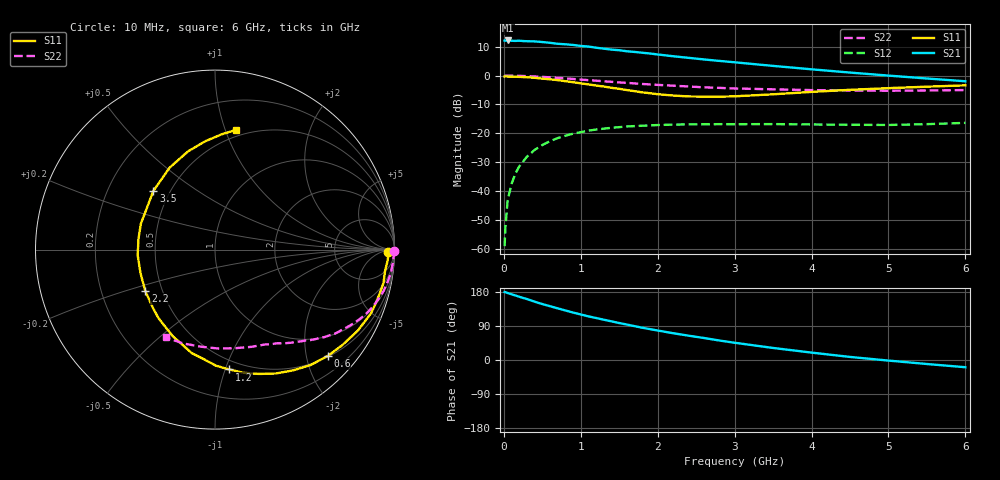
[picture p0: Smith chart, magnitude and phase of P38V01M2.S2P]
! SIEMENS Small Signal Semiconductors
! BFP181
! Si NPN RF Bipolar Junction Transistor in SOT143
! VCE = 8 V  IC = 1.2 mA
! Common Emitter S-Parameters:  March  1996
# GHz  S  MA  R  50
!  f  S11  S21  S12  S22
! GHz  MAG  ANG  MAG  ANG  MAG  ANG  MAG  ANG
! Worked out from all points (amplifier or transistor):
!   36 points, 10 MHz to 6 GHz, reference 50 ohm
!   highest |S21| = 12.2 dB at 50 MHz (marker M1)
!   |S21| within 3 dB of that: start of sweep to 1.347 GHz
!   unconditionally stable (mu >= 1): 3.037 GHz to end of sweep
!   at 250 MHz: K = 0.08, MSG = 20.9 dB, |S12| = -29.8 dB
!   at 1.4 GHz: K = 0.51, MSG = 13.6 dB, |S12| = -18.1 dB
!   at 6 GHz: K = 1.24, MAG = 4.3 dB, |S12| = -16.4 dB
!   S11 on the Smith chart (normalised r, x): 10 MHz: 49, -19; 600 MHz: 0.52, -2.42; 1.2 GHz: 0.42, -1.03; 2.2 GHz: 0.40, -0.23; 3.5 GHz: 0.41, +0.34; 6 GHz: 0.44, +1.09
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0.01  0.9649 -0.8  4.064 179.4  0.0011 88.7  0.9985 -0.3
0.02  0.9657 -1.5  4.037 179.1  0.0023 89.6  0.9978 -0.8
0.05  0.9643 -3.5  4.073 176.7  0.0069 92.5  0.996 -1.8
0.1  0.9548 -7.3  4.028 173.5  0.0132 84.4  0.9956 -3.5
0.2  0.9502 -14.7  4.036 166.9  0.0266 80.3  0.9898 -7.1
0.4  0.9151 -29.5  3.925 153.9  0.0514 70.6  0.9673 -13.7
0.5  0.8868 -36.9  3.824 147.6  0.0625 66.1  0.9504 -17.0
0.6  0.8632 -43.4  3.709 142.0  0.0729 61.8  0.9341 -20.1
0.9  0.7686 -63.9  3.405 125.2  0.0983 50.2  0.8748 -28.0
1.1  0.7041 -77.1  3.192 115.1  0.111 43.4  0.8344 -32.6
1.2  0.6727 -83.2  3.051 110.8  0.1161 40.0  0.817 -34.9
1.5  0.5904 -102.8  2.756 97.5  0.1277 32.6  0.7622 -40.3
1.8  0.5116 -122.8  2.493 85.1  0.1352 26.4  0.7161 -44.9
2.2  0.4517 -149.4  2.168 70.7  0.1412 19.2  0.669 -50.9
2.4  0.4352 -162.6  2.036 64.2  0.1427 16.4  0.6475 -53.7
2.8  0.4306 172.0  1.801 51.5  0.1439 11.9  0.6133 -59.2
3  0.4375 160.7  1.703 45.5  0.1436 9.7  0.5982 -62.0
3.5  0.4741 136.4  1.474 31.8  0.1442 6.1  0.5785 -69.5
4  0.5218 119.0  1.287 19.5  0.1422 3.4  0.5609 -78.3
4.5  0.5673 105.4  1.129 8.1  0.1404 1.8  0.5513 -88.2
5.5  0.6427 86.8  0.891 -10.6  0.1439 2.9  0.552 -108.7
6  0.6782 79.9  0.798 -19.1  0.1515 3.1  0.5616 -119.4
